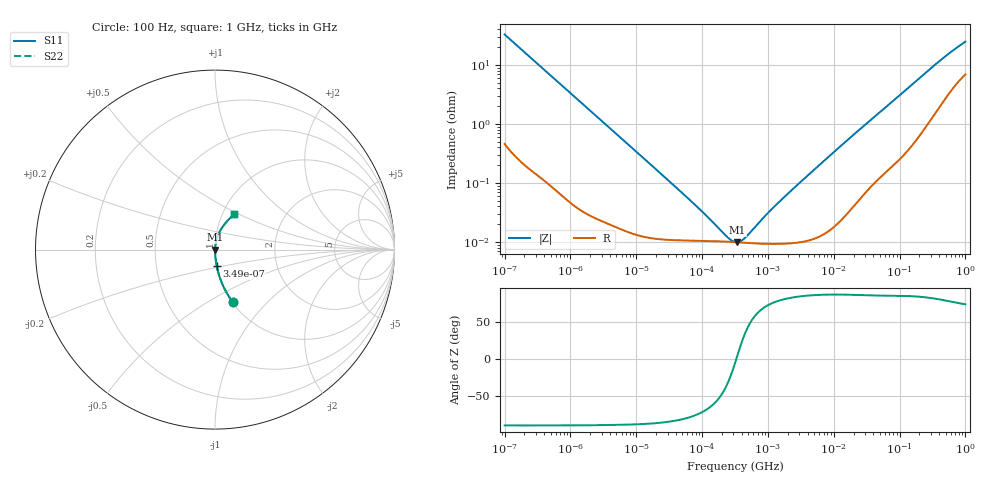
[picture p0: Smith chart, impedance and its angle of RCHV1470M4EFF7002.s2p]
! RCHV1470M4EFF7002  S-PARAMETER MODEL  (AEC-Q200 qualified)
! Model Generated by ELNA Corporation (http://www.ty-top.com)
! Version 1.0
! ELNA Control No. 240229
! Copyright (c) 2024 ELNA CO.,LTD. All Rights Reserved.
! Products Name : CONDUCTIVE POLYMER HYBRID ALUMINUM ELECTROLYTIC CAPACITORS
! Characteristics :
!  Capacitance  :  47uF  ,  Rated voltage  :  63V
!  Operating Temp. Range  :  -55 to +105 degC  ,  Endurance  :  5000hr at 105 degC
!  Dimension D  :  10mm  ,  Dimension L  :  8.7mm
! Frequency Range : 100Hz - 1GHz
! External Node Assignments :
!  1  o---| |---o  2
# MHz S RI R 50
!Freq[MHz].  S11 Real  S11 Imag  S21 Real  S21 Imag  S12 Real  S12 Imag  S22 Real  S22 Imag
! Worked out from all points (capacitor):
!   401 points, 100 Hz to 1 GHz, reference 50 ohm
!   read as one part in series: C = 48.5 uF near 108 Hz
!   lowest |Z| = 9.85 mohm at 342.8 kHz (marker M1)
!   series resonance near 330.8 kHz, so ESL is about 4.8 nH
!   S11 on the Smith chart (normalised r, x): 100 Hz: 1.01, -0.66; 349 Hz: 1.00, -0.19; 1 GHz: 1.14, +0.48
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0.0001  0.1005 -0.2937  0.8995 0.2937  0.8995 0.2937  0.1005 -0.2937
0.000113  0.0809 -0.2662  0.9191 0.2662  0.9191 0.2662  0.0809 -0.2662
0.000176  0.0358 -0.1798  0.9642 0.1798  0.9642 0.1798  0.0358 -0.1798
0.000349  0.0101 -0.0935  0.9899 0.0935  0.9899 0.0935  0.0101 -0.0935
0.000638  0.00339 -0.0517  0.9966 0.0517  0.9966 0.0517  0.00339 -0.0517
0.001488  0.000834 -0.0224  0.9992 0.0224  0.9992 0.0224  0.000834 -0.0224
0.022131  0.000113 -0.00152  0.9999 0.00152  0.9999 0.00152  0.000113 -0.00152
0.090678  0.000104 -0.000347  0.9999 0.000347  0.9999 0.000347  0.000104 -0.000347
0.238506  0.000101 -6.96e-05  0.9999 6.96e-05  0.9999 6.96e-05  0.000101 -6.96e-05
0.280221  9.96e-05 -3.5e-05  0.9999 3.5e-05  0.9999 3.5e-05  9.96e-05 -3.5e-05
0.316228  9.88e-05 -9.47e-06  0.9999 9.47e-06  0.9999 9.47e-06  9.88e-05 -9.47e-06
0.342768  9.82e-05 7.56e-06  0.9999 -7.56e-06  0.9999 -7.56e-06  9.82e-05 7.56e-06
0.386812  9.73e-05 3.34e-05  0.9999 -3.34e-05  0.9999 -3.34e-05  9.73e-05 3.34e-05
0.454465  9.61e-05 6.91e-05  0.9999 -6.91e-05  0.9999 -6.91e-05  9.61e-05 6.91e-05
1.244515  9.23e-05 0.000383  0.9999 -0.000383  0.9999 -0.000383  9.23e-05 0.000383
4.704354  0.000112 0.00156  0.9999 -0.00156  0.9999 -0.00156  0.000112 0.00156
18.51399  0.000397 0.00605  0.9996 -0.00605  0.9996 -0.00605  0.000397 0.00605
69.9842  0.00217 0.0215  0.9978 -0.0215  0.9978 -0.0215  0.00217 0.0215
176.8072  0.00789 0.052  0.9921 -0.052  0.9921 -0.052  0.00789 0.052
395.8221  0.0302 0.1072  0.9698 -0.1072  0.9698 -0.1072  0.0302 0.1072
668.3439  0.0667 0.1573  0.9333 -0.1573  0.9333 -0.1573  0.0667 0.1573
1000  0.1086 0.1983  0.8914 -0.1983  0.8914 -0.1983  0.1086 0.1983
